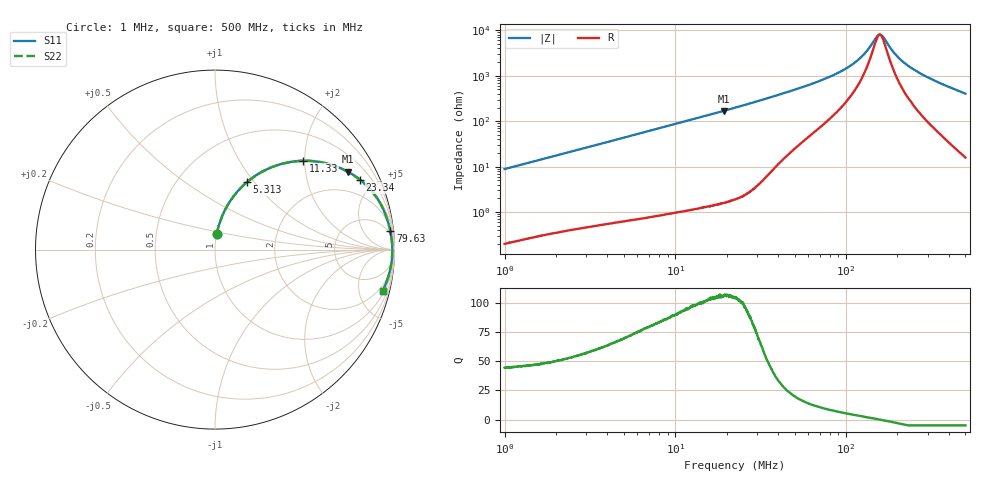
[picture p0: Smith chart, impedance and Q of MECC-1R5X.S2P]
!s-Parameter Generated by FASTRON Sdn. Bhd.
!FASTRON P/N : MECC-1R5X
!Keysight Technologies,E4991B,MY54100416,A.01.15
!Date: Mon Mar 16 14:45:55 2026
!Version  : Rev00 Mon Mar 16 14:45:55 2026
!Data & Calibration Information:
!PortZ  Port1:50+j0  Port2:50+j0
!When reading, reference impedance value at option line is always used.
!Remarks : This data is being provided solely for informational purposes.
!Freq	S11	S21	S12	S22
# Hz S dB R 50
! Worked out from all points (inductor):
!   1601 points, 1 MHz to 500 MHz, reference 50 ohm
!   read as one part in series: L = 1.4 uH near 1.032 MHz
!   highest Q = 106 at 19.22 MHz (marker M1), where L = 1.4 uH
!   self-resonance near 157.7 MHz
!   S11 on the Smith chart (normalised r, x): 1 MHz: 1.00, +0.18; 5.313 MHz: 1.01, +0.92; 11.33 MHz: 1.02, +1.97; 23.34 MHz: 1.04, +4.14; 79.63 MHz: 3, +19; 500 MHz: 1.32, -8.07
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1000000  -21.12 83.7  -0.05 -5.0  -0.05 -5.0  -21.12 83.7
2820919  -12.47 75.2  -0.29 -13.8  -0.29 -13.8  -12.47 75.2
5313102  -7.61 64.6  -0.88 -24.6  -0.88 -24.6  -7.61 64.6
7957584  -4.96 54.9  -1.74 -34.4  -1.74 -34.4  -4.96 54.9
1.133144e7  -3.13 45.1  -2.99 -44.2  -2.99 -44.2  -3.13 45.1
1.921753e7  -1.34 30.5  -5.89 -59.0  -5.89 -59.0  -1.34 30.5
2.236068e7  -1.02 26.7  -6.95 -62.8  -6.95 -62.8  -1.02 26.7
2.333675e7  -0.94 25.7  -7.27 -63.8  -7.27 -63.8  -0.94 25.7
3.605523e7  -0.42 16.5  -10.93 -72.2  -10.93 -72.2  -0.42 16.5
6.307767e7  -0.20 8.4  -16.65 -77.1  -16.65 -77.1  -0.20 8.4
7.963189e7  -0.16 6.0  -19.61 -77.3  -19.61 -77.3  -0.16 6.0
9.89808e7  -0.13 3.9  -23.14 -75.7  -23.14 -75.7  -0.13 3.9
1.16973e8  -0.12 2.5  -26.92 -71.4  -26.92 -71.4  -0.12 2.5
1.309196e8  -0.11 1.5  -30.59 -63.8  -30.59 -63.8  -0.11 1.5
1.494024e8  -0.11 0.4  -36.74 -32.1  -36.74 -32.1  -0.11 0.4
1.553196e8  -0.11 0.1  -38.15 -10.0  -38.15 -10.0  -0.11 0.1
1.633636e8  -0.11 -0.3  -37.62 22.4  -37.62 22.4  -0.11 -0.3
1.77937e8  -0.11 -1.0  -33.40 54.8  -33.40 54.8  -0.11 -1.0
2.070397e8  -0.11 -2.3  -27.44 71.5  -27.44 71.5  -0.11 -2.3
2.543648e8  -0.12 -4.3  -22.45 77.1  -22.45 77.1  -0.12 -4.3
3.403856e8  -0.17 -7.6  -17.56 77.7  -17.56 77.7  -0.17 -7.6
5e8  -0.34 -13.8  -12.46 74.0  -12.46 74.0  -0.34 -13.8
